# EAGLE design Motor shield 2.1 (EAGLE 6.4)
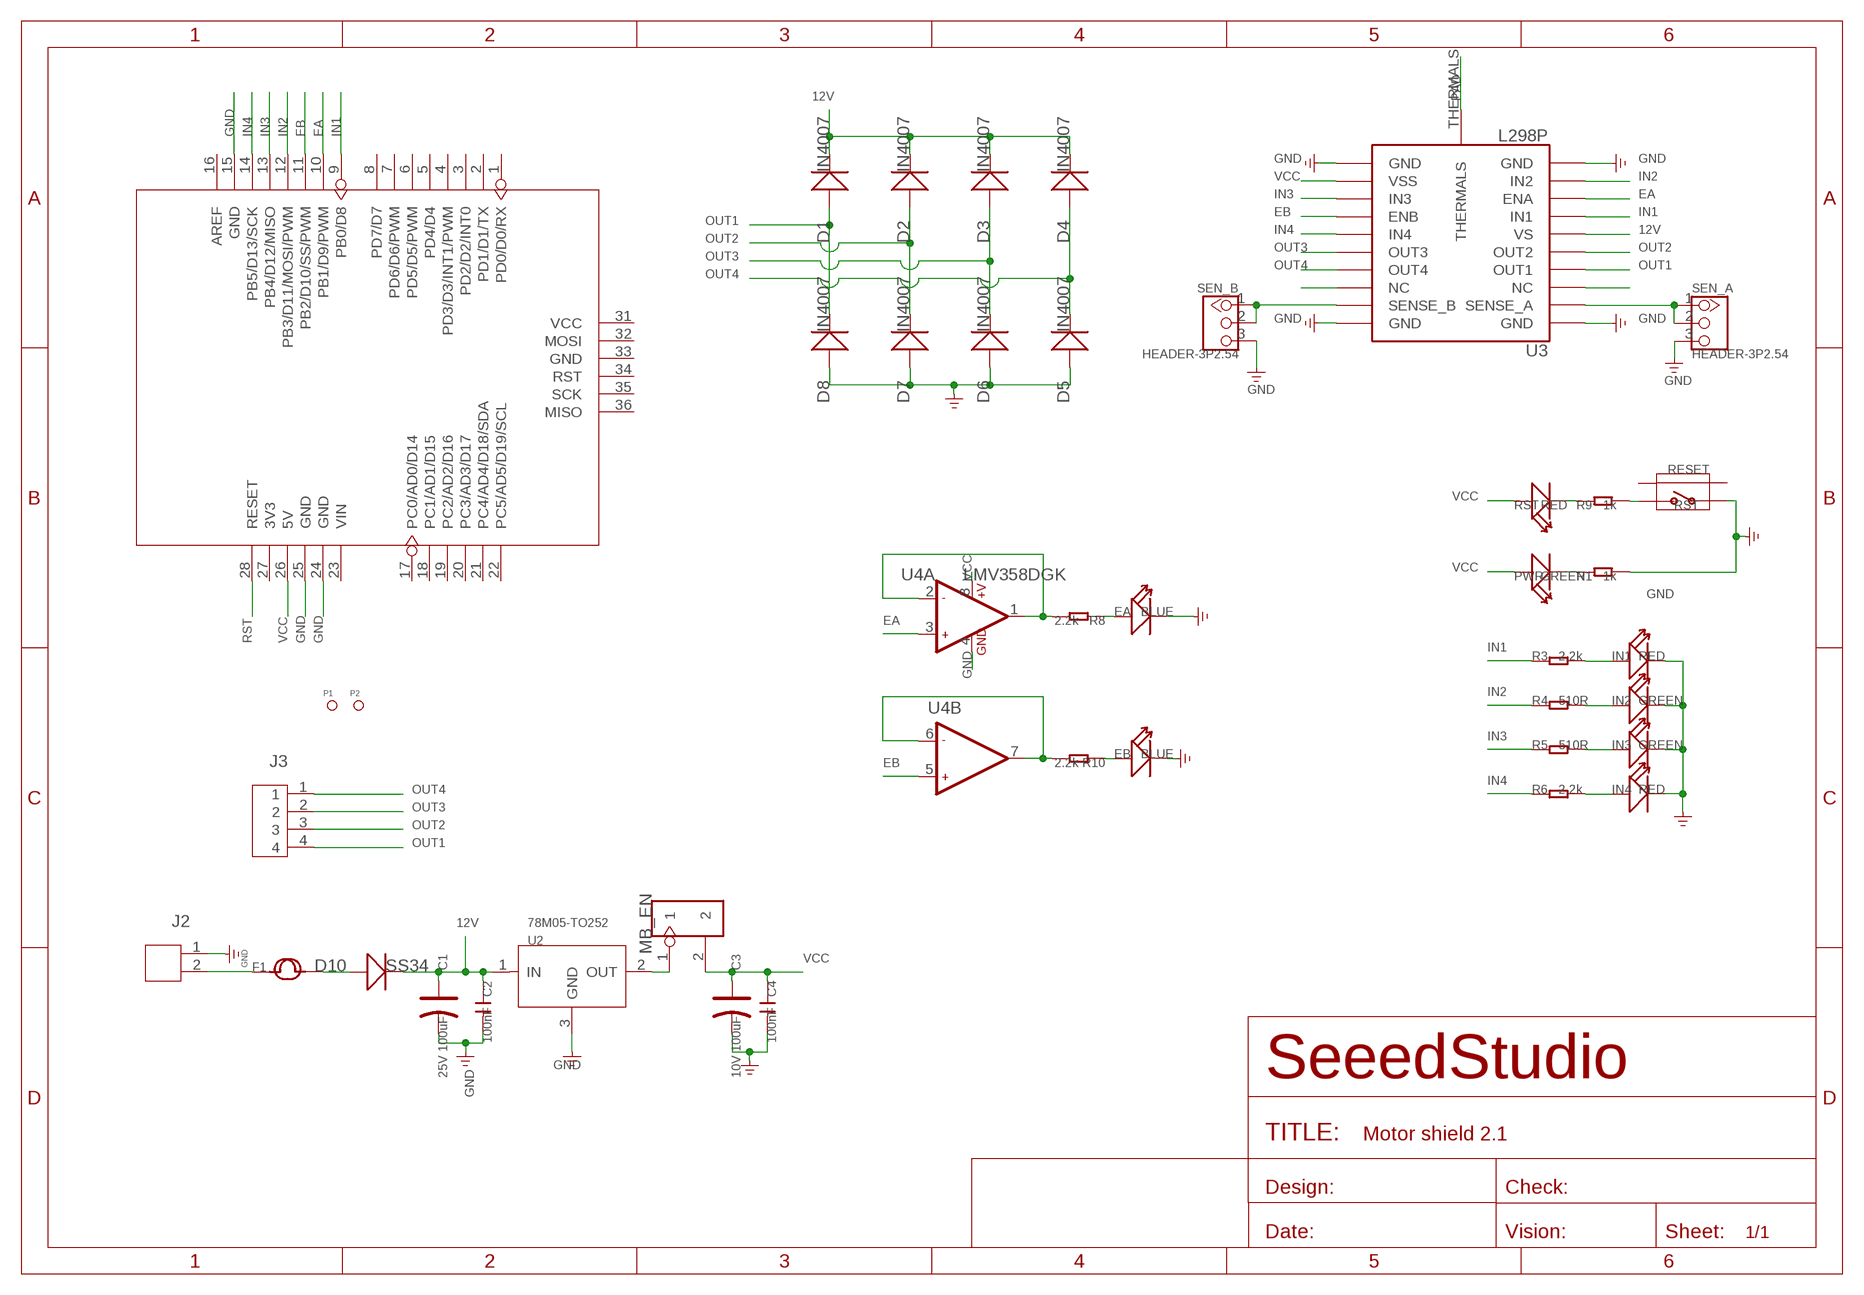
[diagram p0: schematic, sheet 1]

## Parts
C1  25V 100uF  CAP-ELECTRO-D  [ELECTRO-SMD-D-5.6MM]
C2  100nF  C-0603  [C0603]
C3  10V 100uF  CAP-AVX-B  [AVX-B]
C4  100nF  C-0603  [C0603]
D1  IN4007  D'SMA'  [D2010]
D2  IN4007  D'SMA'  [D2010]
D3  IN4007  D'SMA'  [D2010]
D4  IN4007  D'SMA'  [D2010]
D5  IN4007  D'SMA'  [D2010]
D6  IN4007  D'SMA'  [D2010]
D7  IN4007  D'SMA'  [D2010]
D8  IN4007  D'SMA'  [D2010]
D10  SS34  D'DO-214AB'  [DO-214AB]
EA  BLUE  007-LED0603  [D0603]
EB  BLUE  007-LED0603  [D0603]
F1  FUSE'RLD30P250UF'  [0311]
IN1  RED  007-LED0603  [D0603]
IN2  GREEN  007-LED0603  [D0603]
IN3  GREEN  007-LED0603  [D0603]
IN4  RED  007-LED0603  [D0603]
J2  JST-2P-LEADED'3.36'  [2P-3.36-LEADED-7X7]
J3  JST-4P-3.36-LEADED  [4P-3.36-LEADED-7X14]
MB_EN  HEADER-2P-65/35MIL  [2P-2.54-65/35MIL]
P1  PAD-MARK  [ROUND-MARK-1.0]
P2  PAD-MARK  [ROUND-MARK-1.0]
PWR  GREEN  007-LED0603  [D0603]
R1  1k  R-0603  [R0603]
R3  2.2k  R-0603  [R0603]
R4  510R  R-0603  [R0603]
R5  510R  R-0603  [R0603]
R6  2.2k  R-0603  [R0603]
R8  2.2k  R-0603  [R0603]
R9  1k  R-0603  [R0603]
R10  2.2k  R-0603  [R0603]
RESET  BUTTON-4P-REINFORCE'TS-118E'  [4P-SMD-7X3.5X3.5H]
RST  RED  007-LED0603  [D0603]
SEN_A  HEADER-3P2.54  [2.54_1X3P]
SEN_B  HEADER-3P2.54  [2.54_1X3P]
U1  ARDUINO'W/-SILK  [ARDUINO]
U2  78M05-TO252  [TO252]
U3  L298P  [POWERSO-20]
U4  LMV358DGK  [MSOP8]

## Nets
12V: C1.+ C2.1 D1.- D2.- D3.- D4.- D10.2(-) U2.1(IN) U3.P$6(VS)
EA: U1.10(PB1/D9/PWM) U3.P$8(ENA) U4.3(A:+IN1)
EB: U1.11(PB2/D10/SS/PWM) U3.P$14(ENB) U4.5(B:+IN2)
GND: C1.- C2.2 C3.- C4.2 D5.+ D6.+ D7.+ D8.+ EA.- EB.- IN1.- IN2.- IN3.- IN4.- J2.1 R1.2 RESET.1 SEN_A.3 SEN_B.3 U1.15(GND) U1.24(GND) U1.25(GND) U2.3(GND) U3.P$1(GND) U3.P$10(GND) U3.P$11(GND) U3.P$20(GND) U4.4(A:GND)
IN1: R3.1 U1.9(PB0/D8) U3.P$7(IN1)
IN2: R4.1 U1.12(PB3/D11/MOSI/PWM) U3.P$9(IN2)
IN3: R5.1 U1.13(PB4/D12/MISO) U3.P$13(IN3)
IN4: R6.1 U1.14(PB5/D13/SCK) U3.P$15(IN4)
N$1: IN3.+ R5.2
N$2: MB_EN.1 U2.2(OUT)
N$3: PWR.- R1.1
N$4: SEN_A.1 SEN_A.2 U3.P$2(SENSE_A)
N$5: F1.1 J2.2
N$7: U3.P$3(NC)
N$9: D10.1(+) F1.2
N$10: R9.1 RST.-
N$12: EA.+ R8.1
N$14: IN1.+ R3.2
N$15: IN2.+ R4.2
N$16: EB.+ R10.1
N$17: IN4.+ R6.2
N$18: R10.2 U4.6(B:-IN2) U4.7(B:OUT2)
N$19: R8.2 U4.1(A:OUT1) U4.2(A:-IN1)
N$20: SEN_B.1 SEN_B.2 U3.P$19(SENSE_B)
N$23: U3.P$18(NC)
OUT1: D1.+ D8.- J3.4 U3.P$4(OUT1)
OUT2: D2.+ D7.- J3.3 U3.P$5(OUT2)
OUT3: D3.+ D6.- J3.2 U3.P$16(OUT3)
OUT4: D4.+ D5.- J3.1 U3.P$17(OUT4)
PAD: U3.THERMALS
RST: R9.2 RESET.2 U1.28(RESET)
VCC: C3.+ C4.1 MB_EN.2 PWR.+ RST.+ U1.26(5V) U3.P$12(VSS) U4.8(A:+V)
Unconnected: RESET.S1 RESET.S2 U1.1(PD0/D0/RX) U1.2(PD1/D1/TX) U1.3(PD2/D2/INT0) U1.4(PD3/D3/INT1/PWM) U1.5(PD4/D4) U1.6(PD5/D5/PWM) U1.7(PD6/D6/PWM) U1.8(PD7/D7) U1.16(AREF) U1.17(PC0/AD0/D14) U1.18(PC1/AD1/D15) U1.19(PC2/AD2/D16) U1.20(PC3/AD3/D17) U1.21(PC4/AD4/D18/SDA) U1.22(PC5/AD5/D19/SCL) U1.23(VIN) U1.27(3V3) U1.31(VCC) U1.32(MOSI) U1.33(GND) U1.34(RST) U1.35(SCK) U1.36(MISO)

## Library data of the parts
C1 C3 = Discrete:CAP*: Electrolytic Capacitors,Tantalum Capacitors and Super Capacitors
C2 C4 = Discrete:C*: Ceramic Capacitors
D1-D8 D10 = Discrete:D*
EA EB IN1-IN4 PWR RST = Discrete:007-LED*
F1 = Discrete:FUSE
J2 = Connector:JST-2P-LEADED
J3 = Connector:JST-4P-3.36-LEADED
MB_EN = Connector:HEADER-2P
P1 P2 = Discrete:PAD-MARK; PARTNO: DNP
R1 R3-R6 R8-R10 = Discrete:R*
RESET = Discrete:BUTTON-4P-REINFORCE: TS-1188E http://www.best-dz.com/?thread-374-2.html
SEN_A SEN_B = Connector:HEADER-3P
U1 = moudle:ARDUINO
U2 = IC:78M05: 0.5A Three Terminal Positive Voltage Regulators
U3 = IC:L298: Dual Full-Bridge Driver http://www.sandorobotics.com/attachments/l298motores.pdf
U4 = IC:LMV358: General purpose LOW Voltage, Rail-to-Rail Output Amplifiers http://www.fairchildsemi.com/ds/LM/LMV358.pdf

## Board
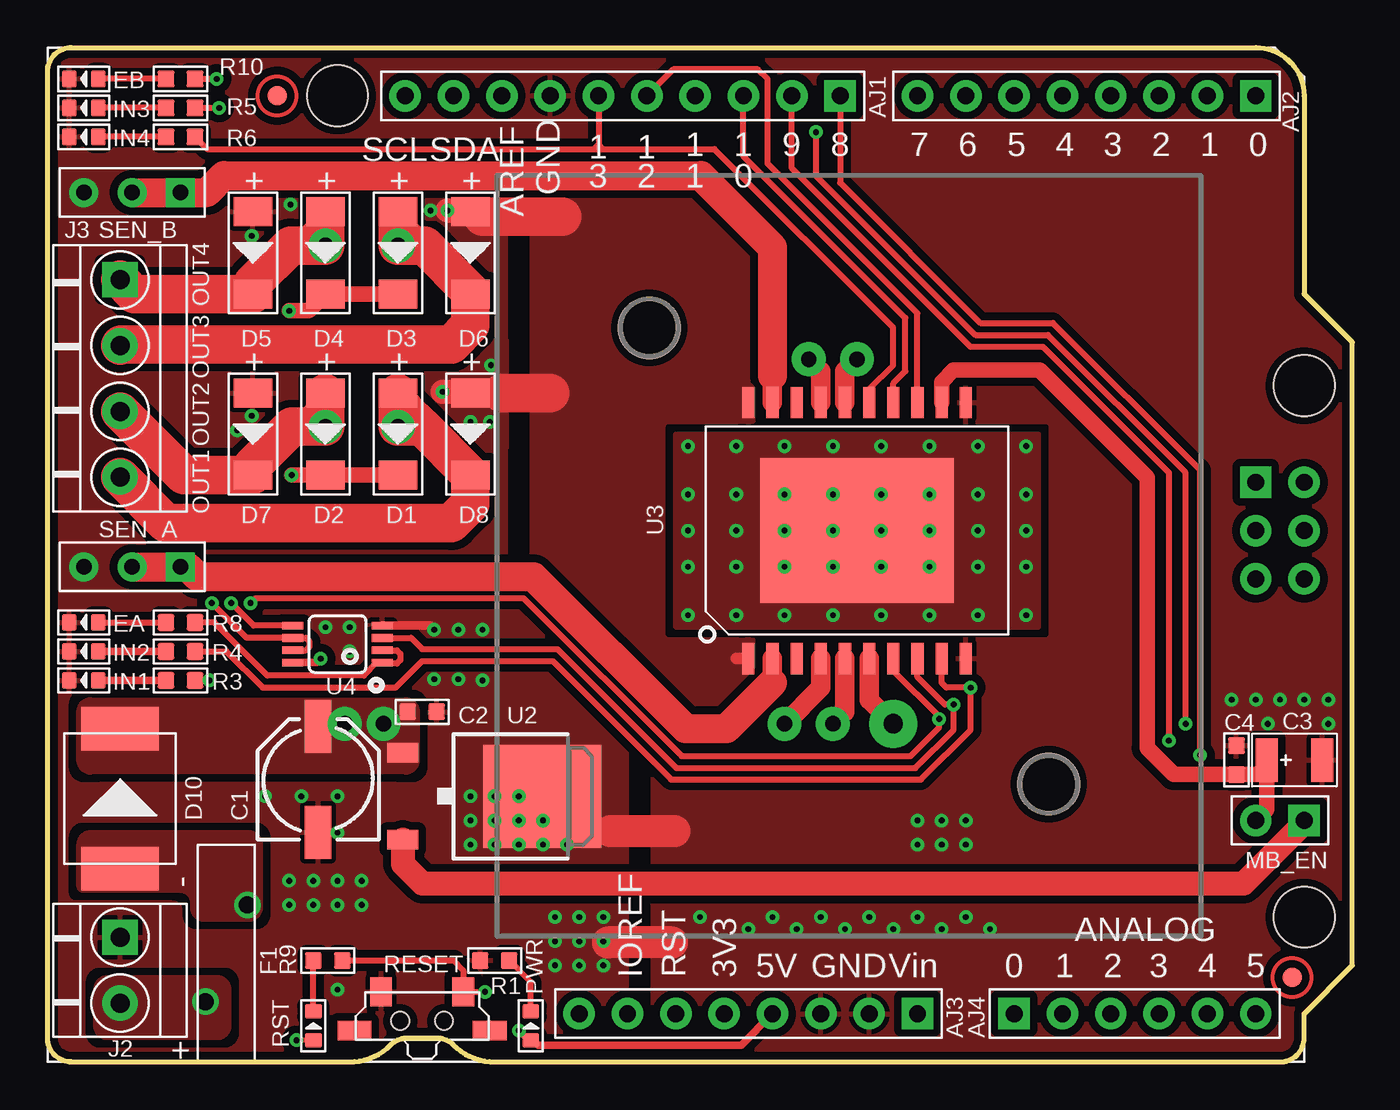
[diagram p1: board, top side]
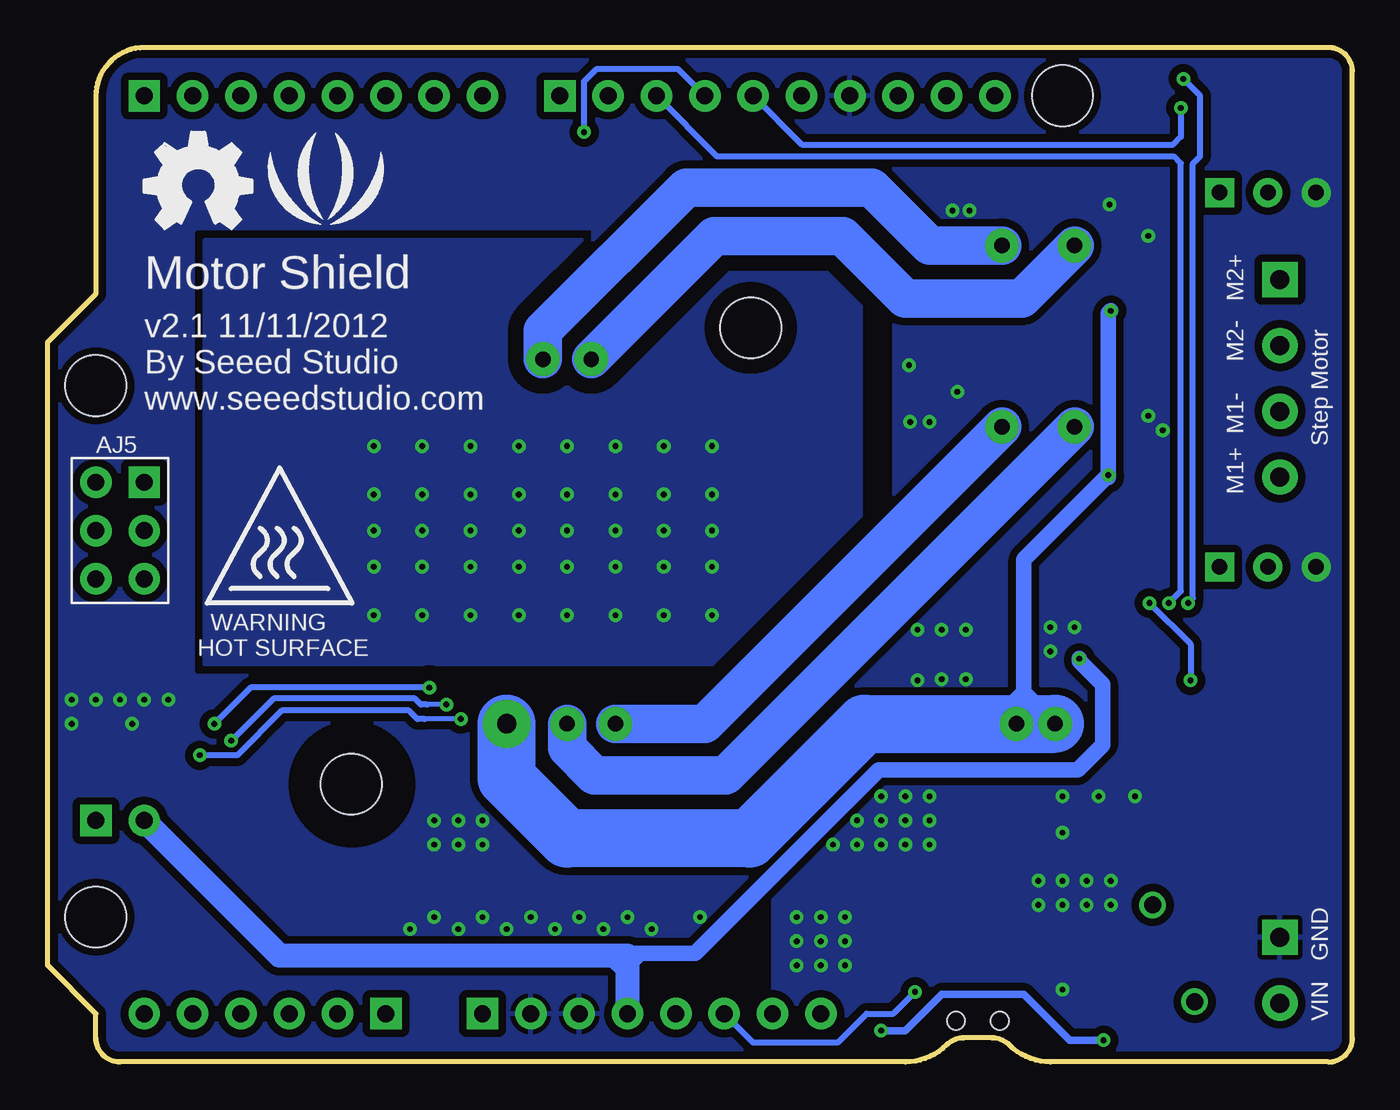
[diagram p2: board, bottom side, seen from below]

Size 68.58 x 53.34 mm. Coordinates in mm from the lower left corner, seen from the top.
Outline: 1.27,0 15.88,0 arc45 18.04,0.9 arc-45 18.94,1.27 20.43,1.27 arc-45 21.33,0.9 arc45 23.5,0 64.77,0 arc90 66.04,1.27 66.04,2.54 68.58,5.08 68.58,37.85 66.04,40.39 66.04,50.8 arc90 63.5,53.34 1.27,53.34 arc90 0,52.07 0,1.27 arc90 1.27,0
Copper layers (1*16): Top 0.035mm / dielectric 1.5mm / Bottom 0.035mm
Design rules "default *": minimum track width 8mil, minimum drill 12mil, track to track 8mil, track to pad 8mil, pad to pad 8mil, via to via 8mil, smd to smd 0mil, copper to edge 10mil, drill to drill 8mil, minimum pad ring 10mil, minimum via ring 8mil, stop-mask expansion 4mil, vias tented up to drill 100mil, thermal gap 10mil
Holes 3.2 mm at 31.62,38.6 52.62,14.6
tRestrict: 3 lines
bRestrict: area 49.7,11.7 to 55.5,17.5; 3 lines

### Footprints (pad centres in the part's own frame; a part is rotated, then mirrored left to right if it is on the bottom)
ELECTRO-SMD-D-5.6MM = smd 2.794 x 1.397: + 2.794,0; - -2.794,0
C0603 = smd 0.889 x 0.889: 1 -0.762,0; 2 0.762,0
AVX-B = smd 1.143 x 2.286: + -1.46,0; - 1.46,0
D2010 = smd 1.524 x 2.032: + -2.159,0; - 2.159,0
DO-214AB = smd 2.286 x 4.064: 1 -3.683,0; 2 3.683,0
D0603 = smd 0.762 x 0.889: + -0.762,0; - 0.762,0
0311 = drill 0.889 pad 1.397: 1 -2.54,1.1; 2 2.54,-1.1
2P-3.36-LEADED-7X7 = drill 1 pad 1.85 square: 1 -1.73,0 | drill 1 pad 1.85: 2 1.73,0
4P-3.36-LEADED-7X14 = drill 1 pad 1.85 square: 1 -5.19,0 | drill 1 pad 1.85: 2 -1.73,0; 3 1.73,0; 4 5.19,0
2P-2.54-65/35MIL = drill 0.889 pad 1.651 square: 1 0,1.27 | drill 0.889 pad 1.651: 2 0,-1.27
ROUND-MARK-1.0 = smd 1.016 x 1.016: P$1 0,0
R0603 = smd 0.889 x 0.889: 1 -0.762,0; 2 0.762,0
4P-SMD-7X3.5X3.5H = smd 1.143 x 1.524: 1 -2.159,1.524; 2 2.159,1.524 | smd 1.778 x 1.016: S1 -3.556,-0.508; S2 3.556,-0.508 | hole 0.95: -1.15,0; 1.15,0
2.54_1X3P = drill 0.813 pad 1.524 square: 1 0,2.54 | drill 0.813 pad 1.524: 2 0,0; 3 0,-2.54
ARDUINO = drill 0.889 pad 1.651 square: 1 63.5,50.8; 9 41.656,50.8; 17 50.8,2.54; 23 45.72,2.54; 36 63.5,30.48 | drill 0.889 pad 1.651: 2 60.96,50.8; 3 58.42,50.8; 4 55.88,50.8; 5 53.34,50.8; 6 50.8,50.8; 7 48.26,50.8; 8 45.72,50.8; 10 39.116,50.8; 11 36.576,50.8; 12 34.036,50.8; 13 31.496,50.8; 14 28.956,50.8; 15 26.416,50.8; 16 23.876,50.8; 18 53.34,2.54; 19 55.88,2.54; 20 58.42,2.54; 21 60.96,2.54; 22 63.5,2.54; 24 43.18,2.54; 25 40.64,2.54; 26 38.1,2.54; 27 35.56,2.54; 28 33.02,2.54; 29 21.336,50.8; 30 18.796,50.8; 31 66.04,30.48; 32 66.04,27.94; 33 66.04,25.4; 34 63.5,25.4; 35 63.5,27.94; 37 30.48,2.54; 38 27.94,2.54 | hole 3.2: 15.24,50.8; 66.04,35.56; 66.04,7.62
TO252 = smd 1.016 x 1.651: 1 -2.286,-4.826; 2 2.286,-4.826 | smd 5.4 x 6.2: 3 0,2.5
POWERSO-20 = smd 1.651 x 0.635: P$1 -6.731,5.715; P$2 -6.731,4.445; P$3 -6.731,3.175; P$4 -6.731,1.905; P$5 -6.731,0.635; P$6 -6.731,-0.635; P$7 -6.731,-1.905; P$8 -6.731,-3.175; P$9 -6.731,-4.445; P$10 -6.731,-5.715; P$11 6.731,-5.715; P$12 6.731,-4.445; P$13 6.731,-3.175; P$14 6.731,-1.905; P$15 6.731,-0.635; P$16 6.731,0.635; P$17 6.731,1.905; P$18 6.731,3.175; P$19 6.731,4.445; P$20 6.731,5.715 | smd 7.62 x 10.16: THERMALS 0,0
MSOP8 = smd 0.4 x 1.1: 1 -0.975,-2.35; 2 -0.325,-2.35; 3 0.325,-2.35; 4 0.975,-2.35; 5 0.975,2.35; 6 0.325,2.35; 7 -0.325,2.35; 8 -0.975,2.35

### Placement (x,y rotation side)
C1  14.22,14.86 90 top
C2  19.68,18.41 0 top
C3  65.53,15.88 0 top
C4  62.48,15.88 90 top
D1  18.41,33.02 270 top
D2  14.61,33.02 270 top
D3  18.41,42.55 270 top
D4  14.61,42.55 270 top
D5  10.79,42.55 270 top
D6  22.23,42.55 270 top
D7  10.79,33.02 270 top
D8  22.23,33.02 270 top
D10  3.81,13.84 90 top
EA  1.91,23.11 180 top
EB  1.91,51.69 180 top
F1  9.4,5.71 90 top
IN1  1.91,20.07 180 top
IN2  1.91,21.59 180 top
IN3  1.91,50.16 180 top
IN4  1.91,48.64 180 top
J2  3.81,4.83 270 top
J3  3.81,35.94 270 top
MB_EN  64.77,12.7 270 top
P1  12.06,50.8 0 top
P2  65.41,4.45 0 top
PWR  25.4,1.91 90 top
R1  23.5,5.33 180 top
R3  6.99,20.07 180 top
R4  6.99,21.59 180 top
R5  6.99,50.16 180 top
R6  6.99,48.64 180 top
R8  6.99,23.11 0 top
R9  14.73,5.33 0 top
R10  6.99,51.69 0 top
RESET  19.68,2.16 0 top
RST  13.97,1.91 90 top
SEN_A  4.45,26.04 270 top
SEN_B  4.45,45.72 270 top
U1  0,0 0 top
U2  23.5,13.97 270 top
U3  42.55,27.94 90 top
U4  15.24,21.97 90 top
U$15  [LOGO_SILK]  53.98,45.72 0 bottom
U$16  [OSHW_FILLX200_NOTEXT]  63.5,43.81 0 bottom

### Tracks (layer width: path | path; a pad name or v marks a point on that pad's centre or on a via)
12V  (via drill 0.3 pad 0.64, 0.81 pad 1.78, 1.02 pad 2.54)
  Top 0.813: v12.83,30.86 D2.- D1.- | D3.- D4.- 13.72,39.5 v12.7,39.5
  Top 1.016: U3.P$6 43.18,19.05 v44.45,17.78
  Bottom 0.813: v12.83,30.86 12.83,39.37 v12.7,39.5 | 12.83,30.73 v12.83,30.86 | 17.27,19.43 17.27,26.42 v12.83,30.86 | 17.27,19.43 16.64,18.8 | 17.27,19.43 17.91,18.8 | 17.27,19.43 17.27,18.42 arc45 17.46,17.98 v17.65,17.78
  Bottom 3.048: v44.45,17.78 44.45,14.92 41.29,11.76 31.68,11.76 25.65,17.78 v17.65,17.78 v15.62,17.78
  pour Top (isolate 0.254, no thermals): 2.29,19.05 18.8,19.05 arc-90 19.43,18.41 19.43,15.88 arc-90 18.8,15.24 2.29,15.24 arc-90 1.65,15.88 1.65,18.41 arc-90
EA  (via drill 0.3 pad 0.64)
  Top 0.305: U3.P$8 45.72,20.23 47.16,18.8 v47.62,18.8 47.62,17.47 45.62,15.46 33.05,15.46 26.8,21.72 24.51,21.72 19.68,21.72 19.11,22.3 U4.3 | v58.93,16.89 58.93,30.99 52.32,37.59 48.51,37.59 39.12,46.99 U1.10
  Bottom 0.254: v47.62,18.8 48.64,18.8
  Bottom 0.305: 48.64,18.8 48.96,18.8 49.28,19.11 56.71,19.11 v58.93,16.89
EB  (via drill 0.3 pad 0.64)
  Top 0.305: U3.P$14 44.45,35.69 45.09,36.32 45.09,39.12 36.58,47.62 U1.11 | U4.5 10.84,22.95 v9.65,24.13
  Bottom 0.305: U1.11 33.4,47.62 9.4,47.62 9.02,47.24 9.02,24.77 v9.65,24.13
GND  (via drill 0.3 pad 0.64)
  Top 0.457: U4.4 20.11,22.95 v20.32,22.73
  Top 0.61: U3.P$1 36.2,21.21
  Top 1.016: D6.+ 26.42,44.7
  Top 1.27: v21.02,44.77 22.16,44.77 D6.+ | v20.77,35.24 22.42,35.24 22.48,35.18
  Top 1.524: D8.+ 23.88,35.18
  Top 1.676: 32.96,12.13 29.59,12.13 | 32.83,6.29 29.46,6.29
  Top 2.032: 22.86,44.45 27.05,44.45 | 23.88,35.18 26.42,35.18
  other vias: 22.23,13.97 22.23,11.43 24.77,11.43 24.77,13.97 27.3,11.43 24.77,12.7 22.23,12.7 11.43,13.97 13.34,13.97 15.24,13.97 15.24,12.06 13.97,9.53 38.1,7.62 40.64,7.62 43.18,7.62 23.24,33.66 23.3,36.64 12.76,45.09 10.73,43.43 10.73,33.97 23.5,13.97 23.5,12.7 23.5,11.43 26.04,11.43 26.04,12.7 21.59,22.73 20.32,20.13 21.59,20.13 22.86,20.07 14.61,22.86 15.88,21.59 22.86,22.73 27.94,5.08 29.21,5.08 34.29,7.62 15.24,3.81 12.7,8.26 16.51,9.53 15.24,9.53 12.7,9.53 13.97,8.26 20.13,44.77 22.23,33.66 26.67,5.08 15.24,8.26 16.51,8.26 27.94,6.35 27.94,7.62 29.21,7.62 29.21,6.35 26.67,6.35 26.67,7.62 15.88,22.86 36.83,6.99 39.37,6.99 41.91,6.99 45.72,12.7 46.99,12.7 48.26,12.7 48.26,11.43 46.99,11.43 45.72,11.43 9.97,33.21 44.45,6.99 45.72,7.62 46.99,6.99 48.26,7.62 49.53,6.99 62.23,19.05 63.5,19.05 64.77,19.05 66.04,19.05 67.31,19.05 67.31,17.78 64.14,17.78
  pour Top (no thermals): 21.34,17.14 29.21,17.14 29.21,10.79 21.34,10.79
  pour Top (isolate 0.254, rank 6): 0,60.33 3.17,60.33 3.17,57.15 0,57.15
  pour Top (isolate 0.406, rank 6): 0,53.34 68.58,53.34 68.58,0 0,0
  pour Bottom (isolate 0.406, rank 6): 0,53.34 68.58,53.34 68.58,0 0,0
  pour Top (isolate 0.254, no thermals): 35.56,22.23 37.08,22.23 37.08,20.72 36.43,20.07 35.56,20.07
  pour Top (isolate 0.254, no thermals): 35.94,35.81 36.72,35.81 37.08,35.45 37.08,33.66 35.94,33.66
  pour Top (isolate 0.254, no thermals): 19.94,45.34 23.62,45.34 23.62,43.18 21.72,43.18 20.57,44.32 19.94,44.32
  pour Top (isolate 0.254, no thermals): 19.94,36.2 21.84,36.2 23.62,37.97 24.13,37.97 24.13,32.26 22.99,32.26 19.94,35.31
  pour Top (isolate 0.254, no thermals): 0.76,27.18 3.05,27.18 3.05,24.89 0.64,24.89 0.64,27.18
  pour Bottom (isolate 0.254, no thermals): 0.76,27.18 3.05,27.18 3.05,24.89 0.64,24.89 0.64,27.18
  pour Bottom (isolate 0.254, no thermals): 0.76,46.86 3.05,46.86 3.05,44.58 0.64,44.58 0.64,46.86
  pour Top (isolate 0.254, no thermals): 0.76,46.86 3.05,46.86 3.05,44.58 0.64,44.58 0.64,46.86
IN1  (via drill 0.3 pad 0.64)
  Top 0.305: U3.P$7 44.45,20.57 46.86,18.16 v46.86,18.03 46.86,17.59 45.36,16.08 33.32,16.08 25.02,24.38 10.92,24.38 v10.67,24.13 | U1.9 41.66,46.23 49.02,38.86 52.83,38.86 60.58,31.11 v60.58,16.13
  Top 0.406: R3.1 v8.51,20.07
  Bottom 0.254: v46.86,18.03 48.77,18.03
  Bottom 0.305: 48.77,18.03 49.15,18.03 49.59,18.48 56.26,18.48 58.61,16.13 v60.58,16.13 | v10.67,24.13 8.51,21.97 v8.51,20.07
IN2  (via drill 0.3 pad 0.64)
  Top 0.305: U3.P$9 46.99,19.94 47.24,19.68 v48.51,19.68 48.51,17.46 45.9,14.85 32.78,14.85 26.54,21.08 19.68,21.08 18.29,19.68 11.3,19.68 9.4,21.59 R4.1 | v40.39,48.9 40.39,46.61 48.77,38.23 52.58,38.23 59.82,30.99 v59.82,17.78
  Bottom 0.305: v48.51,19.68 57.91,19.68 v59.82,17.78 | U1.12 35.43,52.2 39.75,52.2 40.39,51.56 v40.39,48.9
IN3  (via drill 0.3 pad 0.64)
  Top 0.305: U3.P$13 45.72,39.37 37.85,47.24 37.85,51.69 37.34,52.2 32.89,52.2 U1.13 | R5.1 v9.02,50.16
  Bottom 0.305: U1.13 28.93,48.24 9.42,48.24 9.02,48.64 v9.02,50.16
IN4
  Top 0.305: U3.P$15 43.18,35.37 44.44,36.63 44.44,38.62 35.05,48.01 29.21,48.01 | 28.7,48.01 8.38,48.01 R6.1 | 28.7,48.01 29.21,48.01 | U1.14 28.96,48.26 | 28.96,48.26 29.21,48.01 | 28.96,48.26 28.7,48.01
  Top 0.406: R6.1 7.87,48.64
N$1
  Top 0.305: R5.2 IN3.+
N$2
  Top 1.27: U2.2 18.67,10.41 19.71,9.38 62.84,9.38 66.04,12.57 MB_EN.1
N$3
  Top 0.305: PWR.- 25.4,4.19 R1.1
N$4
  Top 1.016: U3.P$2 38.1,19.94
  Top 1.524: SEN_A.2 SEN_A.1 7.37,26.04 7.87,25.53 25.53,25.53 33.53,17.53 35.69,17.53 38.1,19.94
N$5
  pour Top (isolate 0.254, no thermals): 9.53,3.81 9.53,1.91 arc-90 8.89,1.27 3.17,1.27 arc-90 2.54,1.91 2.54,3.81 arc-90 3.17,4.45 8.89,4.45 arc-90
N$9
  pour Top (isolate 0.254, no thermals): 2.29,12.06 10.54,12.06 arc-90 11.18,11.43 11.18,8.13 arc-90 10.54,7.49 8.26,7.49 arc-90 7.62,8.13 7.62,8.38 arc90 6.99,9.02 1.91,9.02 arc-90 1.65,9.27 1.65,11.43 arc-90
N$10
  Top 0.305: RST.- R9.1
N$12
  Top 0.305: EA.+ R8.1
N$14
  Top 0.406: IN1.+ R3.2
N$15
  Top 0.406: IN2.+ R4.2
N$16
  Top 0.305: R10.1 EB.+
N$17
  Top 0.305: R6.2 IN4.+
N$18  (via drill 0.3 pad 0.64)
  Top 0.305: R10.2 v8.89,51.69 | U4.7 13.58,21.65 13.77,21.84 13.77,22.1 13.58,22.3 U4.6 11.5,22.3 10.47,22.3 v8.64,24.13
  Bottom 0.305: v8.89,51.69 8,50.8 8,47.62 8.38,47.24 8.38,24.38 v8.64,24.13
N$19
  Top 0.305: U4.2 18.36,21.65 18.54,21.46 18.54,21.14 18.36,20.95 17.63,20.95 U4.1 17.31,21 16.64,20.32 11.56,20.32 8.76,23.11 R8.2
N$20
  Top 1.016: 38.1,36.07 U3.P$19
  Top 1.524: SEN_B.2 SEN_B.1 8.38,45.72 9.27,46.61 34.33,46.61 38.1,42.84 38.1,36.07
OUT1  (via drill 0.81 pad 1.78)
  Top 1.016: U3.P$4 40.64,19.68 v38.73,17.78
  Top 2.032: 19.68,33.4 v18.41,33.4 D1.+ | 19.68,33.4 D8.- 22.23,29.34 21.23,28.34 6.22,28.34 J3.4 | 19.68,33.4 18.8,34.29
  Bottom 2.032: v38.73,17.78 34.04,17.78 v18.41,33.4
OUT2  (via drill 0.81 pad 1.78)
  Top 1.016: U3.P$5 41.91,18.41 v41.27,17.78
  Top 2.032: 14.61,34.16 v14.61,33.4 12.83,33.4 10.79,31.37 D7.- 7.16,30.86 J3.3 | D2.+ 14.61,34.16 | 14.61,34.16 13.97,33.53
  Bottom 2.032: v14.61,33.4 32.93,15.08 39.84,15.08 41.27,16.51 v41.27,17.78
OUT3  (via drill 0.81 pad 1.78)
  Top 1.016: U3.P$16 41.91,36.32 v42.55,36.96
  Top 1.422: D3.+ 18.41,44.2
  Top 2.032: v18.41,42.93 18.54,42.93 | 18.54,42.93 19.18,42.93 | 19.18,42.93 19.82,42.93 22.23,40.52 D6.- 22.23,38.73 21.21,37.72 3.86,37.72 J3.2 | 18.41,43.69 19.18,42.93 | 18.41,44.2 18.41,43.05 18.54,42.93
  Bottom 2.032: v42.55,36.96 42.55,38.45 35.02,45.97 25.27,45.97 22.23,42.93 v18.41,42.93
OUT4  (via drill 0.81 pad 1.78)
  Top 1.016: U3.P$17 40.64,36.32 v40.01,36.96 | D4.+ 14.61,44.2
  Top 2.032: v14.61,42.93 14.61,43.69 13.84,42.93 | 13.84,42.93 12.78,42.93 10.79,40.94 D5.- 4.55,40.39 J3.1 | 13.84,42.93 v14.61,42.93 | 14.61,44.2 v14.61,42.93
  Bottom 2.032: v14.61,42.93 17.39,40.15 23.51,40.15 26.78,43.42 33.55,43.42 v40.01,36.96
PAD  (via drill 0.3 pad 0.64)
  other vias: 33.66,32.38 51.44,32.38 51.44,29.84 48.9,32.38 46.35,32.38 43.81,32.38 41.27,32.38 38.73,32.38 36.2,32.38 48.9,29.84 46.35,29.84 43.81,29.84 41.27,29.84 38.73,29.84 36.2,29.84 33.66,29.84 33.66,26.04 36.2,26.04 36.2,23.5 33.66,23.5 38.73,26.04 38.73,23.5 41.27,23.5 41.27,26.04 43.81,26.04 43.81,23.5 46.35,23.5 46.35,26.04 48.9,26.04 48.9,23.5 51.44,23.5 51.44,26.04 51.44,27.94 48.9,27.94 46.35,27.94 43.81,27.94 41.27,27.94 38.73,27.94 36.2,27.94 33.66,27.94
  pour Top (isolate 0.254, no thermals): 33.02,33.02 52.07,33.02 52.07,22.86 33.02,22.86
  pour Bottom (isolate 0.813, no thermals): 24.77,43.18 60.33,43.18 60.33,20.95 24.77,20.95
RST  (via drill 0.3 pad 0.64)
  Top 0.305: v22.99,3.68 RESET.2 21.84,4.83 21.34,5.33 R9.2
  Bottom 0.305: U1.28 31.5,1.02 27.05,1.02 25.53,2.54 24.13,2.54 v22.99,3.68
VCC  (via drill 0.3 pad 0.64)
  Top 0.254: RST.+ v13.08,1.14
  Top 0.305: PWR.+ 25.27,1.14 v24.77,1.65
  Top 0.406: PWR.+ 25.53,1.14 25.78,0.89 36.45,0.89 U1.26 | U4.8 14.14,21 v14.35,21.21
  Top 0.813: U3.P$12 46.99,35.76 47.6,36.37 52.15,36.37 57.78,30.73 57.78,16.51 59.18,15.11 C4.1 63.63,15.11 64.01,15.49 64.01,15.81 C3.+ 64.07,13.27 MB_EN.2
  Bottom 0.406: v13.08,1.14 14.86,1.14 17.27,3.56 21.59,3.56 23.5,1.65 v24.77,1.65
  Bottom 0.813: v14.35,21.21 14.35,21.08 13.13,19.86 13.13,16.68 14.44,15.37 24.89,15.37 34.54,5.71 36.83,5.71 37.47,5.71 | 37.47,5.71 38.1,5.08 | 37.47,5.71 38.35,5.71
  Bottom 1.27: U1.26 38.1,4.95 | MB_EN.2 56.39,5.59 38.73,5.59 | 38.1,4.95 38.1,5.08 38.1,5.59 38.73,5.59 | 38.1,4.95 38.73,5.59

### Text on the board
tPlace: AJ1 | AJ2 | SCL | SDA | + | + | + | + | AREF | OUT4 | OUT3 | + | + | + | + | OUT2 | OUT1 | - | IOREF | AJ3 | AJ4 | +
bPlace: Motor Shield | M2+ | v2.1 11/11/2012 | M2- | By Seeed Studio | www.seeedstudio.com | M1- | Step Motor | AJ5 | M1+ | WARNING / HOT SURFACE | GND | VIN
